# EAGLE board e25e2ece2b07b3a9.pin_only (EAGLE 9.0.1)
REV: B

Size 68.58 x 53.34 mm. Coordinates in mm from the lower left corner, seen from the top.
Outline: 64.52,53.34 66.04,51.82 66.04,40.39 68.58,37.85 68.58,5.08 66.04,2.54 66.04,1 arc-90 65.04,0 1,0 arc-90 0,1 0,14.99 1.27,16.26 1.27,21.21 0,22.48 0,52.34 arc-90 1,53.34 64.52,53.34
Copper layers (1*16): Top 0.035mm / dielectric 1.5mm / Bottom 0.035mm
Design rules "adafruit *": minimum track width 8mil, minimum drill 15.5mil, track to track 8mil, track to pad 8mil, pad to pad 8mil, via to via 8mil, smd to smd 8mil, copper to edge 10mil, drill to drill 8mil, minimum pad ring 10mil, minimum via ring 8mil, stop-mask expansion 2mil, vias tented up to drill 20mil, thermal gap 10mil
Holes 3.2 mm at 66.04,35.56 66.04,7.62 15.24,50.8 13.97,2.54

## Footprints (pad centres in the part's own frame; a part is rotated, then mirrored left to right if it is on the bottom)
1X06_OVALWAVE = drill 0.8 pad 1.5 long: 1 -6.35,0; 2 -3.81,0; 3 -1.27,0; 4 1.27,0; 5 3.81,0; 6 6.35,0
0805-NO = smd 1.24 x 1.5: 1 -0.95,0; 2 0.95,0
0603-NO = smd 1.075 x 1: 1 -0.85,0; 2 0.85,0
SOD-123 = smd 1.4 x 1.4: A 1.85,0; C -1.85,0
R1206 = smd 1.6 x 1.803: 1 -1.422,0; 2 1.422,0
FIDUCIAL_1MM = smd 1 x 1: 1 0,0
SOLDERJUMPER_CLOSEDWIRE = smd 1.168 x 1.6: 1 -0.762,0; 2 0.762,0 | smd 0.635 x 0.203: WIRE 0,0
SOT23-5 = smd 0.69 x 0.99: 1 -0.95,-1.29; 2 0,-1.29; 3 0.95,-1.29; 4 0.95,1.3; 5 -0.95,1.3
2X03_ROUND_70MIL = drill 0.9 pad 1.778: 1 -2.54,-1.27; 2 -2.54,1.27; 3 0,-1.27; 4 0,1.27; 5 2.54,-1.27; 6 2.54,1.27
1X10_OVALWAVE = drill 0.8 pad 1.5 long: 1 -11.43,0; 2 -8.89,0; 3 -6.35,0; 4 -3.81,0; 5 -1.27,0; 6 1.27,0; 7 3.81,0; 8 6.35,0; 9 8.89,0; 10 11.43,0
1X08_OVALWAVE = drill 0.8 pad 1.5 long: 1 -8.89,0; 2 -6.35,0; 3 -3.81,0; 4 -1.27,0; 5 1.27,0; 6 3.81,0; 7 6.35,0; 8 8.89,0
1X01_ROUND = drill 1 pad 1.676: 1 0,0
CHIPLED_0805_NOOUTLINE = smd 1.2 x 1.2: A 0,-1.05; C 0,1.05
INDUCTOR_1007 = smd 1.016 x 2.2: P$1 -1.127,0; P$2 1.127,0
LED3535 = smd 1 x 0.85: 1 -1.75,0.875; 2 -1.75,-0.875; 3 1.75,-0.875; 4 1.75,0.875
PANASONIC_D = smd 3.556 x 1.4: + 2.654,0; - -2.654,0
RESPACK_4X0603 = smd 0.45 x 0.9: 1 -1.3,-0.85; 2 -0.4,-0.85; 3 0.4,-0.85; 4 1.3,-0.85; 5 1.3,0.85; 6 0.4,0.85; 7 -0.4,0.85; 8 -1.3,0.85
EVQ-Q2 = smd 3.2 x 1.2: A -3.4,-2; A' 3.4,-2; B -3.4,2; B' 3.4,2
SPDT_SMT_SSSS811101 = smd 0.7 x 1.5: A -2.25,1.75; B 0.75,1.75; C 2.25,1.75 | smd 1 x 0.8: SUP1 -3.65,1.1; SUP2 -3.65,-1.1; SUP3 3.65,1.1; SUP4 3.65,-1.1 | hole 0.9: -1.5,0; 1.5,0
SOT-23 = smd 0.787 x 0.889: 1 0.025,-1.016; 2 -0.94,1.016; 3 0.991,1.016
SOT223-R = smd 1.3 x 1.3: 1 -2.3,-3.05; 2 0,-3.05; 3 2.3,-3.05 | smd 3.6 x 1.3: 4 0,3.05
SOT23-DBV = smd 0.55 x 1.2: 1 -0.95,-1.3; 2 0,-1.3; 3 0.95,-1.3; 4 0.95,1.3; 5 -0.95,1.3
SOIC8_208MIL = smd 0.6 x 2.2: 1 -1.905,-3.315; 2 -0.635,-3.315; 3 0.635,-3.315; 4 1.905,-3.315; 5 1.905,3.315; 6 0.635,3.315; 7 -0.635,3.315; 8 -1.905,3.315
PQFN64-1 = smd 0.7 x 0.22: 1 -4.45,3.75; 2 -4.45,3.25; 3 -4.45,2.75; 4 -4.45,2.25; 5 -4.45,1.75; 6 -4.45,1.25; 7 -4.45,0.75; 8 -4.45,0.25; 9 -4.45,-0.25; 10 -4.45,-0.75; 11 -4.45,-1.25; 12 -4.45,-1.75; 13 -4.45,-2.25; 14 -4.45,-2.75; 15 -4.45,-3.25; 16 -4.45,-3.75; 33 4.45,-3.75; 34 4.45,-3.25; 35 4.45,-2.75; 36 4.45,-2.25; 37 4.45,-1.75; 38 4.45,-1.25; 39 4.45,-0.75; 40 4.45,-0.25; 41 4.45,0.25; 42 4.45,0.75; 43 4.45,1.25; 44 4.45,1.75; 45 4.45,2.25; 46 4.45,2.75; 47 4.45,3.25; 48 4.45,3.75 | smd 0.22 x 0.7: 17 -3.75,-4.45; 18 -3.25,-4.45; 19 -2.75,-4.45; 20 -2.25,-4.45; 21 -1.75,-4.45; 22 -1.25,-4.45; 23 -0.75,-4.45; 24 -0.25,-4.45; 25 0.25,-4.45; 26 0.75,-4.45; 27 1.25,-4.45; 28 1.75,-4.45; 29 2.25,-4.45; 30 2.75,-4.45; 31 3.25,-4.45; 32 3.75,-4.45; 49 3.75,4.45; 50 3.25,4.45; 51 2.75,4.45; 52 2.25,4.45; 53 1.75,4.45; 54 1.25,4.45; 55 0.75,4.45; 56 0.25,4.45; 57 -0.25,4.45; 58 -0.75,4.45; 59 -1.25,4.45; 60 -1.75,4.45; 61 -2.25,4.45; 62 -2.75,4.45; 63 -3.25,4.45; 64 -3.75,4.45 | smd 4.7 x 4.7: EXP 0,0
2X05_1.27MM_BOX_POSTS = smd 0.76 x 2.6: 1 -2.54,-2.15; 2 -2.54,2.15; 3 -1.27,-2.15; 4 -1.27,2.15; 5 0,-2.15; 6 0,2.15; 7 1.27,-2.15; 8 1.27,2.15; 9 2.54,-2.15; 10 2.54,2.15 | hole 1: -1.905,0; 1.905,0
4UCONN_20329_V2 = smd 1 x 2: BASE@1 -0.75,-2; BASE@2 0.75,-2 | smd 0.4 x 1.35: D+ 0,0.775; D- -0.65,0.775; GND 1.3,0.775; ID 0.65,0.775; VBUS -1.3,0.775 | drill 0.8 pad 1.143 offset: SPRT@1 -3.3,0.9; SPRT@2 3.3,0.9 | drill 0.9 pad 2.413 square: SPRT@3 -3.6,-1.9; SPRT@4 3.6,-1.9 | hole 0.7: -1.95,0; 1.95,0
XTAL3215 = smd 1.1 x 1.9: P$1 1.2,0; P$2 -1.2,0
DCJACK_2MM_PTH = drill 1 pad 2.7 long: GND 7.35,0; GNDBREAK 10.75,-4.8; PWR 13.6,0

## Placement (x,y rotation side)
AD  20609  [1X06_OVALWAVE]  57.15,2.54 0 top
C1  10uF  [0805-NO]  26.78,25.27 225 top
C2  0.1uF  [0805-NO]  22.99,13.84 180 top
C3  10uF  [0805-NO]  26.54,10.03 0 top
C4  .1u  [0603-NO]  41.78,17.14 270 top
C5  22pF  [0603-NO]  36.83,18.16 270 top
C6  .1u  [0603-NO]  27.92,7.33 90 top
C7  22pF  [0603-NO]  37.72,15.11 180 top
C8  .1u  [0603-NO]  27.55,22.41 135 top
C9  1uF  [0603-NO]  29.37,26.78 135 top
C10  .1u  [0603-NO]  29.94,29.05 315 top
C11  .1u  [0603-NO]  31.66,21.12 45 top
C12  0.1uF  [0603-NO]  16.89,23.11 0 top
C13  0.1uF  [0603-NO]  26.54,11.81 180 top
C14  .1u  [0603-NO]  42.28,20.5 90 top
C15  .1u  [0603-NO]  37.54,37.72 270 top
C16  .1u  [0603-NO]  47.14,32.49 180 top
C17  0.1uF  [0603-NO]  14.35,45.49 90 top
D1  MBR120  [SOD-123]  13.74,13.39 180 top
F2  500mA  [R1206]  8.76,32.38 270 top
FB2  FERRITE  [0805-NO]  1.78,44.83 270 top
FD1  FIDUCIAL_1MM  [FIDUCIAL_1MM]  10.92,49.28 0 top
FD2  FIDUCIAL_1MM  [FIDUCIAL_1MM]  66.16,4.55 0 top
FD3  FIDUCIAL_1MM  [FIDUCIAL_1MM]  22.91,3.28 0 top
GROUND1  [SOLDERJUMPER_CLOSEDWIRE]  7.11,44.7 180 bottom
IC3  74LVC1G125D  [SOT23-5]  13.03,29.03 90 top
ICSP  3x2 M  [2X03_ROUND_70MIL]  64.64,27.94 270 top
IOH  20611  [1X10_OVALWAVE]  30.23,50.8 0 top
IOL  20610  [1X08_OVALWAVE]  54.61,50.8 0 top
JP1  [1X01_ROUND]  5.46,13.72 0 top
L  RED  [CHIPLED_0805_NOOUTLINE]  3.68,31.62 90 top
L1  10uH  [INDUCTOR_1007]  29.39,23.8 315 top
LED1  WS2812B3535  [LED3535]  11.3,41.15 180 top
ON  GREEN  [CHIPLED_0805_NOOUTLINE]  3.56,24.64 270 top
PC1  47uF/25V  [PANASONIC_D]  19.08,10.29 90 top
PC2  47uF+/6.3V+  [PANASONIC_D]  21.59,18.26 180 top
POWER  20610  [1X08_OVALWAVE]  36.83,2.54 0 top
R1  100K  [RESPACK_4X0603]  17.78,29.72 90 top
R2  1K  [RESPACK_4X0603]  7.24,27.3 270 top
R3  10K  [0603-NO]  16.02,45.48 90 top
R4  1K  [0603-NO]  64.14,13.59 270 top
R5  10K  [0603-NO]  56.13,35.18 180 top
R7  10K  [0603-NO]  14.1,6.86 90 top
R11  330R  [0603-NO]  17.32,32.79 0 top
RESET  EVQQ 6mm  [EVQ-Q2]  6.35,49.4 180 top
RXLED  YELLOW  [CHIPLED_0805_NOOUTLINE]  3.56,29.46 270 top
SJ1  AREF_3V  [SOLDERJUMPER_CLOSEDWIRE]  17.27,23.37 180 bottom
SW1  [SPDT_SMT_SSSS811101]  2.92,18.8 270 top
T2  DMP3098L-7  [SOT-23]  13.46,10.29 180 top
TR1  DMP3098L-7  [SOT-23]  12.7,24.31 90 top
TXLED  YELLOW  [CHIPLED_0805_NOOUTLINE]  3.56,26.92 270 top
U1  NCP1117ST50T3G  [SOT223-R]  12.88,18.44 90 top
U2  AP2112K-3.3  [SOT23-DBV]  24.77,7.37 270 top
U3  SPI Flash  [SOIC8_208MIL]  55.24,29.46 180 top
U$1  ATSAMD51J  [PQFN64-1]  38.3,28.1 135 top
U$23  [METROM4_REVF_TOP]  0,0 0 top
U$27  [METROM4_REVF_BOT]  68.58,0 0 bottom
X2  2x5 0.05" SWD  [2X05_1.27MM_BOX_POSTS]  61.34,19.3 180 top
X3  20329  [4UCONN_20329_V2]  4.32,38.1 270 top
X4  32.768  [XTAL3215]  38.73,17.78 90 top
X5  2.1mm  [DCJACK_2MM_PTH]  -3.3,7.75 0 top

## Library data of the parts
AD C1-C17 D1 FB2 GROUND1 ICSP IOH IOL JP1 L L1 LED1 ON PC1 PC2 POWER R1-R5 R7 R11 RESET RXLED SJ1 SW1 TXLED U1 U3 U$1 X2 X3 X5 = microbuilder
F2 = adafruit
FD1-FD3 = microbuilder; BOM: EXCLUDE
IC3 = 74xx-little-de
T2 = zetex; OC_FARNELL: unknown; OC_NEWARK: unknown
TR1 = Transistors; CASE: SOT23; MONTHLY_USAGE: _____; PART_NUMBER: PMV48XP; PRICE: _____; SUPPLIER: _____; TYPE: Transistor
U2 = SmartPrj
U$23 U$27 = silks
X4 = adafruit2

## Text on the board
tNames: SCL | SDA | AREF | GND | 1 | ANALOG IN | IOREF | RESET | 3V3 | 5V | GND | VIN | A0 | A1 | A2 | A3 | A4 | A5
214bmp: D:/SmartProjects/Snc/a4_bn_logo2.bmp

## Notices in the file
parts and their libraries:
microbuilder: This work is placed in the public domain, and may be freely used for commercial and non-commercial work with the following conditions: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
